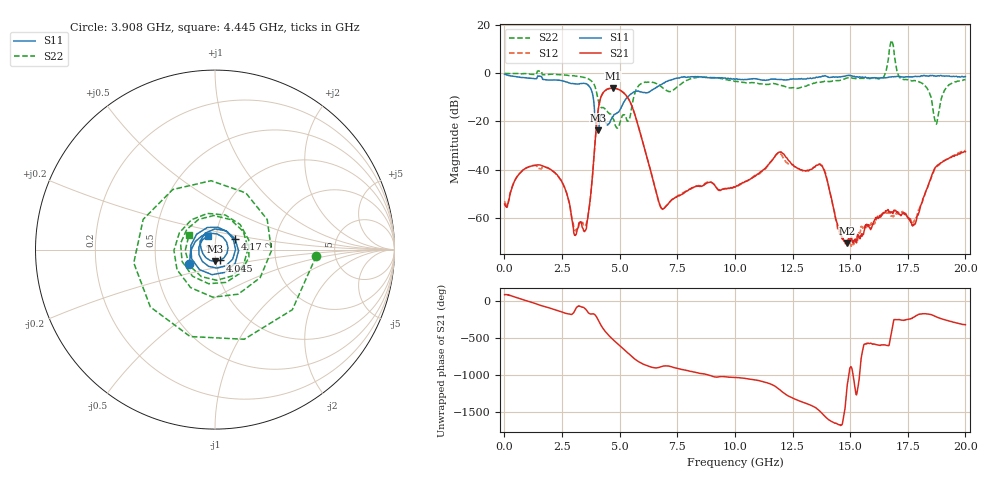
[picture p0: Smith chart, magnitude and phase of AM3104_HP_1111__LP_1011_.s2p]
!Created with skrf (http://scikit-rf.org).
# Hz S RI R 50.0
!freq ReS11 ImS11 ReS21 ImS21 ReS12 ImS12 ReS22 ImS22
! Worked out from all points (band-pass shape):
!   1601 points, 10 MHz to 20 GHz, reference 50 ohm
!   highest |S21| = -6.11 dB at 4.708 GHz (marker M1); lowest = -70.6 dB at 14.87 GHz (marker M2)
!   |S21| within 3 dB of the highest: 4.222 GHz to 5.276 GHz (1.054 GHz wide, 22.2 % of centre)
!   lowest |S11| = -23.6 dB at 4.058 GHz (marker M3), VSWR 1.14, Z = 49.5 - j6.54 ohm
!   |S11| at or under -10 dB: 3.855 GHz to 5.323 GHz (1.468 GHz wide, 32 % of centre)
!   |S22| runs from -22.8 to 13.6 dB; largest |S21 - S12| = 0.044
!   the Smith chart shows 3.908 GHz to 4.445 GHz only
!   S11 on the Smith chart (normalised r, x): 3.908 GHz: 0.74, -0.12; 4.045 GHz: 1.05, -0.13; 4.17 GHz: 1.24, +0.15; 4.445 GHz: 0.92, +0.14
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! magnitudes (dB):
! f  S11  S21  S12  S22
! 10 MHz  -0.4  -54.3  -53.1  -0.1
! 1.584 GHz  -1.3  -38.2  -39.7  0.9
! 3.346 GHz  -4.2  -62.0  -61.9  -1.5
! 3.596 GHz  -4.6  -61.4  -60.9  -2.1
! 3.908 GHz  -15.7  -31.8  -32.0  -5.0
! 4.045 GHz  -23.6  -17.0  -17.0  -10.0
! 4.058 GHz  -23.6  -16.0  -16.1  -10.6
! 4.17 GHz  -17.9  -10.4  -10.4  -13.9
! 4.445 GHz  -21.2  -6.6  -6.7  -15.6
! 4.708 GHz  -18.0  -6.1  -6.2  -18.7
! 5.52 GHz  -8.4  -13.3  -13.3  -14.3
! 6.682 GHz  -5.3  -52.8  -52.9  -4.7
! 10.01 GHz  -2.5  -47.3  -47.3  -3.4
! 11.93 GHz  -2.5  -32.7  -33.0  -4.9
! 13.34 GHz  -2.1  -39.8  -39.7  -4.4
! 13.84 GHz  -1.2  -39.7  -39.3  -3.5
! 14.87 GHz  -1.0  -70.6  -69.4  -2.0
! 16.38 GHz  -1.9  -58.7  -58.4  -2.1
! 16.68 GHz  -1.6  -57.6  -58.0  7.2
! 17.78 GHz  -1.4  -62.9  -61.2  -3.0
! 18.73 GHz  -1.2  -38.8  -39.1  -21.0
! 20 GHz  -1.4  -32.5  -32.1  -2.6
